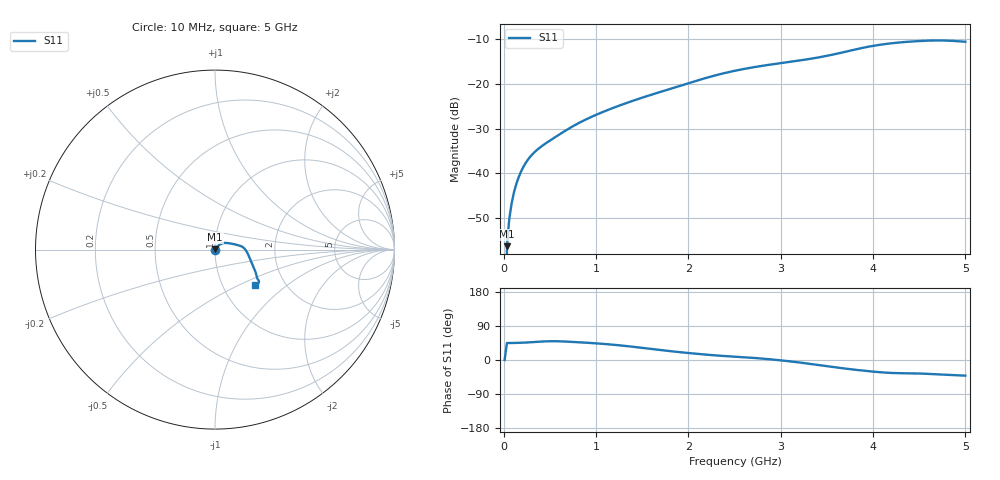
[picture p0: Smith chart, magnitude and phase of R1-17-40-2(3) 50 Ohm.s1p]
!version-1
!date-02.2022
!Test device: КШБА.685111.033
#	GHZ	S	RI	R	50.0
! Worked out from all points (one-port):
!   200 points, 10 MHz to 5 GHz, reference 50 ohm
!   lowest |S11| = -56.2 dB at 35.08 MHz (marker M1), VSWR 1.00, Z = 50.1 + j0.109 ohm
!   |S11| at or under -10 dB: start of sweep to end of sweep
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0.01  0 0
0.0350754  0.00109 0.00108
0.0601508  0.00218 0.00217
0.0852261  0.00326 0.00324
0.110302  0.00431 0.0043
0.135377  0.00533 0.00535
0.160452  0.00632 0.00638
0.185528  0.00727 0.00739
0.210603  0.00817 0.00837
0.260754  0.00979 0.0103
0.33598  0.0117 0.0128
0.436281  0.0138 0.0159
0.636884  0.0188 0.0217
0.787337  0.0241 0.026
0.912714  0.0289 0.0293
1.26377  0.0453 0.036
1.51452  0.0605 0.0373
1.89065  0.0877 0.0338
2.24171  0.1175 0.0274
2.51754  0.1397 0.0212
2.76829  0.157 0.012
3.14442  0.1785 -0.015
3.44533  0.1945 -0.0503
3.77131  0.2158 -0.0995
4.07221  0.2314 -0.1459
4.39819  0.2428 -0.1708
4.6991  0.2415 -0.1879
5  0.2223 -0.1954
